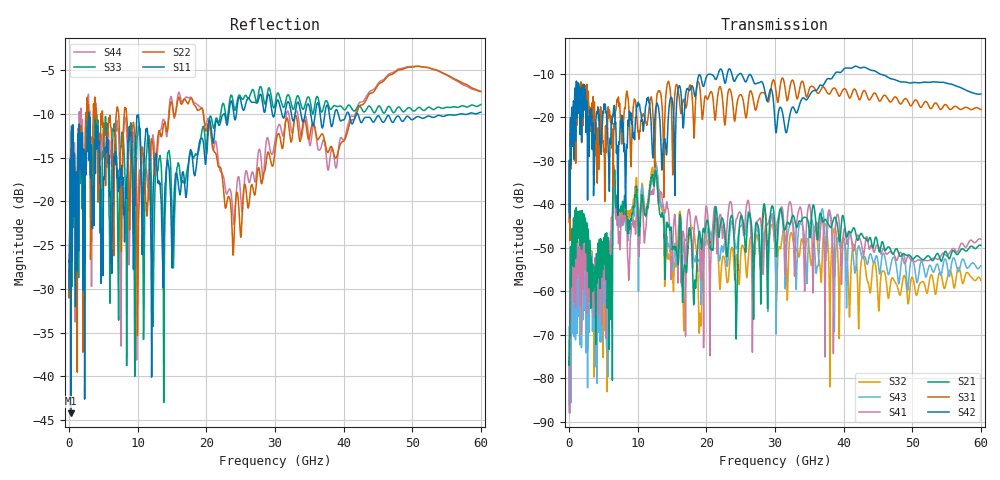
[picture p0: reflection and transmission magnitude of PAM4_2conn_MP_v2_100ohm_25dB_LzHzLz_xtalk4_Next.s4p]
! Info: Touchstone file created by Circ.  Input file=FAB50GbE_2conn_Midplane_Examax_Topo2_v2_100ohm_25dB_LzHzLz.circ
# Hz S RI R 50
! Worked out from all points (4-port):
!   6000 points, 10 MHz to 60 GHz, reference 50 ohm
!   strongest paths, dB at 10 MHz, 15.01 GHz, 30.01 GHz, 45.01 GHz, 60 GHz:
!     S42: -41.8, -15.8, -21.2, -9.7, -14.6
!     S31: -44.1, -24.0, -12.4, -15.7, -18.2
!     S21: -76.1, -50.3, -45.6, -49.5, -49.4
!     S41: -68.2, -53.0, -48.6, -49.5, -48.0
!     S43: -71.3, -54.2, -50.3, -53.3, -54.1
!     S32: -75.2, -53.5, -50.0, -61.9, -57.5
!   lowest |S11| = -44.2 dB at 270 MHz (marker M1), VSWR 1.01, Z = 49.5 + j0.344 ohm
!   |S11| at or under -10 dB: start of sweep to 2.838 GHz; 2.87 GHz to 22.53 GHz (19.66 GHz wide, 155 % of centre); 42.08 GHz to 56.91 GHz (14.83 GHz wide, 30 % of centre)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
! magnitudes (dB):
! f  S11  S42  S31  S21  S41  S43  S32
! 10 MHz  -30.1  -41.8  -44.1  -76.1  -68.2  -71.3  -75.2
! 270 MHz  -44.2  -25.6  -26.5  -54.0  -62.8  -74.8  -64.4
! 12.65 GHz  -14.5  -17.6  -19.1  -32.4  -32.3  -30.6  -30.4
! 19.1 GHz  -12.9  -10.3  -13.8  -47.2  -53.8  -55.1  -65.0
! 19.9 GHz  -15.7  -11.2  -15.1  -45.3  -41.3  -49.0  -46.8
! 28.48 GHz  -9.8  -13.6  -14.4  -40.0  -47.9  -46.1  -41.0
! 60 GHz  -9.8  -14.6  -18.2  -49.4  -48.0  -54.1  -57.5
